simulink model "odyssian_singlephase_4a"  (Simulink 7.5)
settings: Solver=ode23t  StartTime=0.0  StopTime=6  RelTol=1e-6
undefined symbols (not defined in the file or in its folder): dfilt, DiscIntNeverNeededParam
libraries: powerlib x80, powerlib_extras x43, simulink x24, dsparch4 x4
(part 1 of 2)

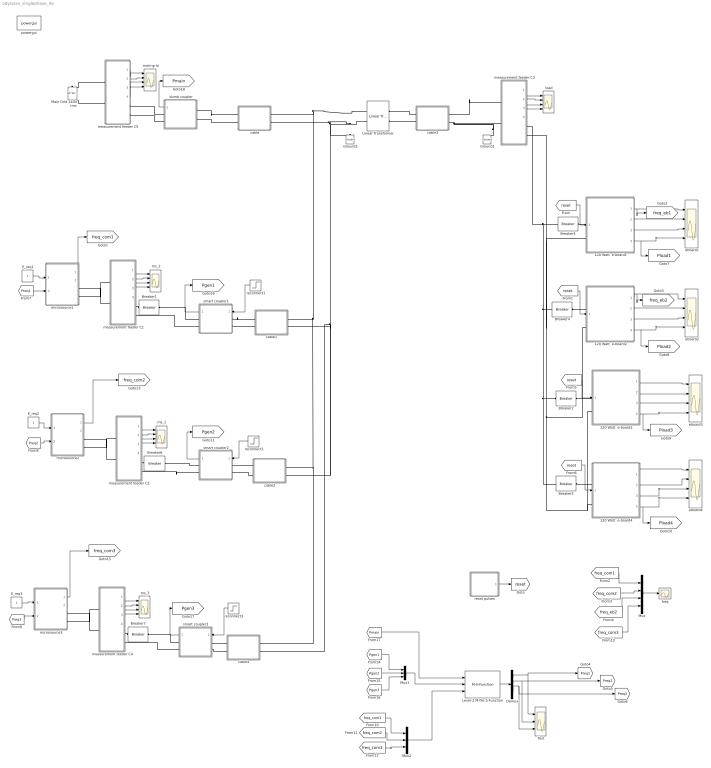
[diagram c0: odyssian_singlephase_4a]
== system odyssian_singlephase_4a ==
  " load" : Scope  NumInputPorts=4
  " main-grid" : Scope  NumInputPorts=4
  " ms_1" : Scope  NumInputPorts=4
  " ms_2" : Scope  NumInputPorts=4
  " ms_3" : Scope  NumInputPorts=4
  120 Watt  e-board1 : Subsystem  mask{tf=100, p=1}
      mask prompts: tf "fault_time"; p "load priority"
  120 Watt  e-board2 : Subsystem  mask{tf=100, p=1}
      mask prompts: tf "fault_time"; p "load priority"
  120 Watt  e-board3 : Subsystem  mask{tf=100, p=1}
      mask prompts: tf "fault_time"; p "load priority"
  120 Watt  e-board4 : Subsystem  mask{tf=100, p=2}
      mask prompts: tf "fault_time"; p "load priority"
  Breaker{1..6} (6 alike) : powerlib/Elements/Breaker  DialogController=POWERSYS.PowerSysDialog  SystemSampleTime=-1  BreakerResistance=0.01  InitialState=1  SnubberResistance=1e6  SnubberCapacitance=inf  SwitchingTimes=[100]  External=off  Measurements=None  MoreParameters=off  NoBreakLoop=off
  Breaker7 : powerlib/Elements/Breaker  DialogController=POWERSYS.PowerSysDialog  SystemSampleTime=-1  BreakerResistance=0.01  InitialState=1  SnubberResistance=1e6  SnubberCapacitance=inf  SwitchingTimes=[3 4.5]  External=off  Measurements=None  MoreParameters=off  NoBreakLoop=off
  Demux : Demux  Outputs=3
  E_req1 : Constant  OutDataType=fixdt(1, 16)  OutScaling=2^0
  E_req2 : Constant  OutDataType=fixdt(1, 16)  OutScaling=2^0
  E_req3 : Constant  OutDataType=fixdt(1, 16)  OutScaling=2^0
  Ground1 : powerlib/Elements/Ground  DialogController=POWERSYS.PowerSysDialog  PhysicalDomain=powersysdomain  SubClassName=unknown  LeftPortType=p1  RightPortType=p1  LConnTagsString=a
  Ground3 : powerlib/Elements/Ground  DialogController=POWERSYS.PowerSysDialog  PhysicalDomain=powersysdomain  SubClassName=unknown  LeftPortType=p1  RightPortType=p1  LConnTagsString=a
  Level-2 M-file S-Function : M-S-Function  FunctionName=Power_Dispatcher
  Linear Transformer : powerlib/Elements/Linear Transformer  DialogController=POWERSYS.PowerSysDialog  PhysicalDomain=powersysdomain  SubClassName=unknown  LeftPortType=p1  RightPortType=p1  LConnTagsString=a|b  RConnTagsString=A|B  UNITS=SI  NominalPower=[ 45e3 , 60 ]  winding1=[240 0.001 1.e-3]  winding2=[120 .001 1.e-3]  ThreeWindings=off  winding3=[3.15e+05 0.7938 0.084225]  RmLm=[1.0804e+06 2866]  Measurements=All voltages and currents  DataType=on
  Main Grid 240V rms : powerlib/Electrical Sources/AC Voltage Source  DialogController=POWERSYS.PowerSysDialog  SystemSampleTime=-1  Amplitude=240*sqrt(2)  Phase=0  Frequency=60  SampleTime=0  Measurements=None
  Mux : Mux
  Mux1 : Mux  Inputs=3
  Mux2 : Mux  Inputs=3
  Test : Scope  NumInputPorts=3
  cable : Subsystem
  cable1 : Subsystem
  cable2 : Subsystem
  cable3 : Subsystem
  cable4 : Subsystem
  dumb coupler : Subsystem
  eboard{1..4} (4 alike) : Scope  NumInputPorts=4
  freq : Scope
  measurement feeder C1 : Subsystem
  measurement feeder C2 : Subsystem
  measurement feeder C3 : Subsystem
  measurement feeder C4 : Subsystem
  measurement feeder C5 : Subsystem
  microsource1 : Subsystem  AncestorBlock=|
      | UWM_blocks/inverter-based
      | DG (simplified)
      | 208V - 15kVA
  microsource2 : Subsystem  AncestorBlock=|
      | UWM_blocks/inverter-based
      | DG (simplified)
      | 208V - 15kVA
  microsource3 : Subsystem  AncestorBlock=|
      | UWM_blocks/inverter-based
      | DG (simplified)
      | 208V - 15kVA
  powergui : powerlib/powergui  Priority=1  SystemSampleTime=-1  SimulationMode=Discrete  SampleTime=50e-5  frequency=60  SPID=off  DisableSnubberDevices=off  DisableRonSwitches=off  DisableVfSwitches=off  SwTol=0  Interpol=off  frequencyindice=0  echomessages=off  HookPort=off  DisplayEquations=off  FunctionMessages=off  EnableUseOfTLC=off  x0status=blocks  RestoreLinks=warning  ResistiveCurrentMeasurement=off  Frange=[0:2:500]  Ylog=off  Xlog=on  ShowGrid=off  save=off  variable=ZData  ZoomFFT=on  StartTime=0.0  cycles=1  DisplayStyle=1  fundamental=60  FreqAxis=off  MaxFrequency=1000  frequencyindicesteady=1  RmsSteady=1  display=off  Ts=0  methode=off
  reconnect1 : Step  Time=.1  SampleTime=0
  reconnect2 : Step  Time=.1  SampleTime=0
  reconnect3 : Step  Time=.1  SampleTime=0
  reset pulses : Subsystem  mask{tpulse=[50 100]}
  smart coupler1 : Subsystem
  smart coupler2 : Subsystem
  smart coupler3 : Subsystem
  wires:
  measurement feeder C3/1(Vm) -> " load"/1
  measurement feeder C3/2(Im) -> " load"/2
  measurement feeder C3/3(PQ) -> " load"/3
  measurement feeder C3/4(RMS (V-I)) -> " load"/4
  120 Watt  e-board1/1(w) -> eboard1/1, [freq_eb1]
  120 Watt  e-board1/2(Irms) -> eboard1/2
  120 Watt  e-board1/3(Vrms) -> eboard1/3
  [reset] -> 120 Watt  e-board1/1(reset)
  120 Watt  e-board2/1(w) -> eboard2/1, [freq_eb2]
  120 Watt  e-board2/2(Irms) -> eboard2/2
  120 Watt  e-board2/3(Vrms) -> eboard2/3
  [reset] -> 120 Watt  e-board2/1(reset)
  Mux/1 -> freq/1
  reset pulses/1(Out1) -> [reset]
  [freq_com1] -> Mux/1
  [freq_com2] -> Mux/2
  [freq_eb2] -> Mux/3
  measurement feeder C5/1(Vm) -> " main-grid"/1
  measurement feeder C5/2(Im) -> " main-grid"/2
  measurement feeder C5/3(PQ) -> " main-grid"/3
  measurement feeder C5/4(RMS (V-I)) -> " main-grid"/4
  measurement feeder C1/1(Vm) -> " ms_2"/1
  measurement feeder C1/2(Im) -> " ms_2"/2
  measurement feeder C1/3(PQ) -> " ms_2"/3
  measurement feeder C1/4(RMS (V-I)) -> " ms_2"/4
  E_req1/1 -> microsource1/1(E_req)
  120 Watt  e-board3/1(w) -> eboard3/1
  120 Watt  e-board3/2(Irms) -> eboard3/2
  120 Watt  e-board3/3(Vrms) -> eboard3/3
  [reset] -> 120 Watt  e-board3/1(reset)
  120 Watt  e-board4/1(w) -> eboard4/1
  120 Watt  e-board4/2(Irms) -> eboard4/2
  [reset] -> 120 Watt  e-board4/1(reset)
  measurement feeder C2/1(Vm) -> " ms_1"/1
  measurement feeder C2/2(Im) -> " ms_1"/2
  measurement feeder C2/3(PQ) -> " ms_1"/3
  measurement feeder C2/4(RMS (V-I)) -> " ms_1"/4
  E_req2/1 -> microsource2/1(E_req)
  reconnect2/1 -> smart coupler2/1(switch)
  measurement feeder C4/1(Vm) -> " ms_3"/1
  measurement feeder C4/2(Im) -> " ms_3"/2
  measurement feeder C4/3(PQ) -> " ms_3"/3
  measurement feeder C4/4(RMS (V-I)) -> " ms_3"/4
  E_req3/1 -> microsource3/1(E_req)
  [Preq2] -> microsource2/2(P_req)
  [Preq3] -> microsource3/2(P_req)
  [Preq1] -> microsource1/2(P_req)
  120 Watt  e-board1/4(Pload) -> eboard1/4, [Pload1]
  120 Watt  e-board2/4(Pload) -> eboard2/4, [Pload2]
  120 Watt  e-board3/4(Pload) -> eboard3/4, [Pload3]
  120 Watt  e-board4/3(Vrms) -> eboard4/3
  120 Watt  e-board4/4(Pload) -> eboard4/4, [Pload4]
  microsource1/1(w) -> [freq_com1]
  microsource2/1(w) -> [freq_com2]
  microsource3/1(w) -> [freq_com3]
  [Pgen2] -> Mux1/2
  smart coupler2/1(Pgen) -> [Pgen2]
  smart coupler1/1(Pgen) -> [Pgen1]
  reconnect1/1 -> smart coupler1/1(switch)
  smart coupler3/1(Pgen) -> [Pgen3]
  reconnect3/1 -> smart coupler3/1(switch)
  dumb coupler/1(Pgen) -> [Pmain]
  [Pmain] -> Level-2 M-file S-Function/1
  [Pgen1] -> Mux1/1
  [Pgen3] -> Mux1/3
  Mux1/1 -> Level-2 M-file S-Function/2
  [freq_com1] -> Mux2/1
  [freq_com2] -> Mux2/2
  [freq_com3] -> Mux2/3
  Mux2/1 -> Level-2 M-file S-Function/3
  Level-2 M-file S-Function/1 -> Demux/1
  Demux/1 -> Test/1, [Preq1]
  Demux/2 -> Test/2, [Preq2]
  Demux/3 -> Test/3, [Preq3]
  [freq_com3] -> Mux/4
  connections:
  Breaker2/RConn1 -- Breaker4/RConn1 -- measurement feeder C3/RConn1 -- Breaker3/RConn1 -- Breaker5/RConn1
  120 Watt  e-board4/LConn2 -- measurement feeder C3/RConn2 -- 120 Watt  e-board1/LConn2 -- 120 Watt  e-board2/LConn2 -- 120 Watt  e-board3/LConn2
  cable3/LConn2 -- Ground1/LConn1 -- measurement feeder C3/LConn2
  120 Watt  e-board1/LConn1 -- Breaker3/LConn1
  120 Watt  e-board2/LConn1 -- Breaker4/LConn1
  measurement feeder C5/RConn1 -- dumb coupler/RConn1
  cable4/LConn1 -- Linear Transformer/LConn1 -- cable/LConn1 -- cable1/LConn1 -- cable2/LConn1
  Linear Transformer/LConn2 -- Ground3/LConn1 -- cable2/LConn2 -- cable4/LConn2 -- cable1/LConn2 -- cable/LConn2
  cable3/LConn1 -- measurement feeder C3/LConn1
  cable3/RConn2 -- Linear Transformer/RConn2
  cable3/RConn1 -- Linear Transformer/RConn1
  measurement feeder C5/LConn1 -- Main Grid 240V rms/RConn1
  measurement feeder C5/LConn2 -- Main Grid 240V rms/LConn1
  measurement feeder C1/LConn1 -- microsource1/RConn1
  Breaker1/RConn1 -- measurement feeder C1/RConn1
  120 Watt  e-board3/LConn1 -- Breaker2/LConn1
  120 Watt  e-board4/LConn1 -- Breaker5/LConn1
  measurement feeder C2/LConn1 -- microsource2/RConn1
  measurement feeder C2/LConn2 -- microsource2/RConn2
  Breaker6/RConn1 -- measurement feeder C2/RConn1
  measurement feeder C4/LConn1 -- microsource3/RConn1
  measurement feeder C4/LConn2 -- microsource3/RConn2
  Breaker7/RConn1 -- measurement feeder C4/RConn1
  measurement feeder C1/LConn2 -- microsource1/RConn2
  cable2/RConn1 -- smart coupler2/LConn1
  cable2/RConn2 -- smart coupler2/LConn2
  smart coupler2/RConn1 -- Breaker6/LConn1
  smart coupler2/RConn2 -- measurement feeder C2/RConn2
  smart coupler1/RConn1 -- Breaker1/LConn1
  smart coupler1/LConn1 -- cable1/RConn1
  smart coupler1/LConn2 -- cable1/RConn2
  smart coupler1/RConn2 -- measurement feeder C1/RConn2
  smart coupler3/RConn1 -- Breaker7/LConn1
  smart coupler3/RConn2 -- measurement feeder C4/RConn2
  smart coupler3/LConn1 -- cable4/RConn1
  smart coupler3/LConn2 -- cable4/RConn2
  measurement feeder C5/RConn2 -- dumb coupler/RConn2
  dumb coupler/LConn1 -- cable/RConn1
  dumb coupler/LConn2 -- cable/RConn2

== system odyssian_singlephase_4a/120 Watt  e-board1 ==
  reset : Inport
  Breaker : powerlib/Elements/Breaker  DialogController=POWERSYS.PowerSysDialog  SystemSampleTime=-1  BreakerResistance=0.01  InitialState=1  SnubberResistance=1e6  SnubberCapacitance=inf  SwitchingTimes="[ 1/60  5/60 ]"  External=on  Measurements=None  MoreParameters=off  NoBreakLoop=off
  Current Measurement : powerlib/Measurements/Current Measurement  DialogController=POWERSYS.PowerSysDialog  SystemSampleTime=-1  PhasorSimulation=off  OutputType=Complex  PSBequivalent=0
  Ground : powerlib/Elements/Ground  DialogController=POWERSYS.PowerSysDialog  PhysicalDomain=powersysdomain  SubClassName=unknown  LeftPortType=p1  RightPortType=p1  LConnTagsString=a
  Product : Product  OutDataType=fixdt(1, 16)  OutScaling=2^0
  Series RLC Load : powerlib/Elements/Series RLC Load  DialogController=POWERSYS.PowerSysDialog  PhysicalDomain=powersysdomain  SubClassName=unknown  LeftPortType=p1  RightPortType=p1  LConnTagsString=a  RConnTagsString=__new0  NominalVoltage=120  NominalFrequency=60  ActivePower=120  InductivePower=0  CapacitivePower=0  Setx0=off  InitialVoltage=0  SetiL0=off  InitialCurrent=0  Measurements=None
  Voltage  Measurement : powerlib/Measurements/Voltage Measurement  DialogController=POWERSYS.PowerSysDialog  SystemSampleTime=-1  PhasorSimulation=off  OutputType=Complex  PSBequivalent=0
  trip : Subsystem  mask{p=p}
      mask prompts: p "priority level"
  A : PMIOPort  Port=1  Side=Left
  C : PMIOPort  Port=2  Side=Left
  w : Outport  OutDataType=fixdt(1, 16)  OutScaling=2^0
  Irms : Outport  Port=2  OutDataType=fixdt(1, 16)  OutScaling=2^0
  Vrms : Outport  Port=3  OutDataType=fixdt(1, 16)  OutScaling=2^0
  Pload : Outport  Port=4  OutDataType=fixdt(1, 16)  OutScaling=2^0
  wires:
  trip/1(w) -> w/1
  Current Measurement/1 -> trip/3(I)
  Voltage  Measurement/1 -> trip/2(V)
  reset/1 -> trip/1(Reset)
  trip/2(trip) -> Breaker/1
  trip/3(Irms) -> Irms/1, Product/1
  trip/4(Vrms) -> Vrms/1, Product/2
  Product/1 -> Pload/1
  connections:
  A/RConn1 -- Current Measurement/LConn1 -- Voltage  Measurement/LConn1
  Voltage  Measurement/LConn2 -- Ground/LConn1
  Current Measurement/RConn1 -- Breaker/LConn1
  Series RLC Load/LConn1 -- Breaker/RConn1
  Series RLC Load/RConn1 -- C/RConn1

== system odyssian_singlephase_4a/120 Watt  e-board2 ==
  reset : Inport
  Breaker : powerlib/Elements/Breaker  DialogController=POWERSYS.PowerSysDialog  SystemSampleTime=-1  BreakerResistance=0.01  InitialState=1  SnubberResistance=1e6  SnubberCapacitance=inf  SwitchingTimes="[ 1/60  5/60 ]"  External=on  Measurements=None  MoreParameters=off  NoBreakLoop=off
  Current Measurement : powerlib/Measurements/Current Measurement  DialogController=POWERSYS.PowerSysDialog  SystemSampleTime=-1  PhasorSimulation=off  OutputType=Complex  PSBequivalent=0
  Ground : powerlib/Elements/Ground  DialogController=POWERSYS.PowerSysDialog  PhysicalDomain=powersysdomain  SubClassName=unknown  LeftPortType=p1  RightPortType=p1  LConnTagsString=a
  Product : Product  OutDataType=fixdt(1, 16)  OutScaling=2^0
  Series RLC Load : powerlib/Elements/Series RLC Load  DialogController=POWERSYS.PowerSysDialog  PhysicalDomain=powersysdomain  SubClassName=unknown  LeftPortType=p1  RightPortType=p1  LConnTagsString=a  RConnTagsString=__new0  NominalVoltage=120  NominalFrequency=60  ActivePower=120  InductivePower=0  CapacitivePower=0  Setx0=off  InitialVoltage=0  SetiL0=off  InitialCurrent=0  Measurements=None
  Voltage  Measurement : powerlib/Measurements/Voltage Measurement  DialogController=POWERSYS.PowerSysDialog  SystemSampleTime=-1  PhasorSimulation=off  OutputType=Complex  PSBequivalent=0
  trip : Subsystem  mask{p=p}
      mask prompts: p "priority level"
  A : PMIOPort  Port=1  Side=Left
  C : PMIOPort  Port=2  Side=Left
  w : Outport  OutDataType=fixdt(1, 16)  OutScaling=2^0
  Irms : Outport  Port=2  OutDataType=fixdt(1, 16)  OutScaling=2^0
  Vrms : Outport  Port=3  OutDataType=fixdt(1, 16)  OutScaling=2^0
  Pload : Outport  Port=4  OutDataType=fixdt(1, 16)  OutScaling=2^0
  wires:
  trip/1(w) -> w/1
  Current Measurement/1 -> trip/3(I)
  Voltage  Measurement/1 -> trip/2(V)
  reset/1 -> trip/1(Reset)
  trip/2(trip) -> Breaker/1
  trip/3(Irms) -> Irms/1, Product/1
  trip/4(Vrms) -> Vrms/1, Product/2
  Product/1 -> Pload/1
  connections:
  A/RConn1 -- Current Measurement/LConn1 -- Voltage  Measurement/LConn1
  Voltage  Measurement/LConn2 -- Ground/LConn1
  Current Measurement/RConn1 -- Breaker/LConn1
  Series RLC Load/LConn1 -- Breaker/RConn1
  Series RLC Load/RConn1 -- C/RConn1

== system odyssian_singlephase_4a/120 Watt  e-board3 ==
  reset : Inport
  Breaker : powerlib/Elements/Breaker  DialogController=POWERSYS.PowerSysDialog  SystemSampleTime=-1  BreakerResistance=0.01  InitialState=1  SnubberResistance=1e6  SnubberCapacitance=inf  SwitchingTimes="[ 1/60  5/60 ]"  External=on  Measurements=None  MoreParameters=off  NoBreakLoop=off
  Current Measurement : powerlib/Measurements/Current Measurement  DialogController=POWERSYS.PowerSysDialog  SystemSampleTime=-1  PhasorSimulation=off  OutputType=Complex  PSBequivalent=0
  Ground : powerlib/Elements/Ground  DialogController=POWERSYS.PowerSysDialog  PhysicalDomain=powersysdomain  SubClassName=unknown  LeftPortType=p1  RightPortType=p1  LConnTagsString=a
  Product : Product  OutDataType=fixdt(1, 16)  OutScaling=2^0
  Series RLC Load : powerlib/Elements/Series RLC Load  DialogController=POWERSYS.PowerSysDialog  PhysicalDomain=powersysdomain  SubClassName=unknown  LeftPortType=p1  RightPortType=p1  LConnTagsString=a  RConnTagsString=__new0  NominalVoltage=120  NominalFrequency=60  ActivePower=120  InductivePower=0  CapacitivePower=0  Setx0=off  InitialVoltage=0  SetiL0=off  InitialCurrent=0  Measurements=None
  Voltage  Measurement : powerlib/Measurements/Voltage Measurement  DialogController=POWERSYS.PowerSysDialog  SystemSampleTime=-1  PhasorSimulation=off  OutputType=Complex  PSBequivalent=0
  trip : Subsystem  mask{p=p}
      mask prompts: p "priority level"
  A : PMIOPort  Port=1  Side=Left
  C : PMIOPort  Port=2  Side=Left
  w : Outport  OutDataType=fixdt(1, 16)  OutScaling=2^0
  Irms : Outport  Port=2  OutDataType=fixdt(1, 16)  OutScaling=2^0
  Vrms : Outport  Port=3  OutDataType=fixdt(1, 16)  OutScaling=2^0
  Pload : Outport  Port=4  OutDataType=fixdt(1, 16)  OutScaling=2^0
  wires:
  trip/1(w) -> w/1
  Current Measurement/1 -> trip/3(I)
  Voltage  Measurement/1 -> trip/2(V)
  reset/1 -> trip/1(Reset)
  trip/2(trip) -> Breaker/1
  trip/3(Irms) -> Irms/1, Product/1
  trip/4(Vrms) -> Vrms/1, Product/2
  Product/1 -> Pload/1
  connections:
  A/RConn1 -- Current Measurement/LConn1 -- Voltage  Measurement/LConn1
  Voltage  Measurement/LConn2 -- Ground/LConn1
  Current Measurement/RConn1 -- Breaker/LConn1
  Series RLC Load/LConn1 -- Breaker/RConn1
  Series RLC Load/RConn1 -- C/RConn1

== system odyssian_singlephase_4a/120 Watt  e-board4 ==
  reset : Inport
  Breaker : powerlib/Elements/Breaker  DialogController=POWERSYS.PowerSysDialog  SystemSampleTime=-1  BreakerResistance=0.01  InitialState=1  SnubberResistance=1e6  SnubberCapacitance=inf  SwitchingTimes="[ 1/60  5/60 ]"  External=on  Measurements=None  MoreParameters=off  NoBreakLoop=off
  Current Measurement : powerlib/Measurements/Current Measurement  DialogController=POWERSYS.PowerSysDialog  SystemSampleTime=-1  PhasorSimulation=off  OutputType=Complex  PSBequivalent=0
  Ground : powerlib/Elements/Ground  DialogController=POWERSYS.PowerSysDialog  PhysicalDomain=powersysdomain  SubClassName=unknown  LeftPortType=p1  RightPortType=p1  LConnTagsString=a
  Product : Product  OutDataType=fixdt(1, 16)  OutScaling=2^0
  Series RLC Load : powerlib/Elements/Series RLC Load  DialogController=POWERSYS.PowerSysDialog  PhysicalDomain=powersysdomain  SubClassName=unknown  LeftPortType=p1  RightPortType=p1  LConnTagsString=a  RConnTagsString=__new0  NominalVoltage=120  NominalFrequency=60  ActivePower=120  InductivePower=0  CapacitivePower=0  Setx0=off  InitialVoltage=0  SetiL0=off  InitialCurrent=0  Measurements=None
  Voltage  Measurement : powerlib/Measurements/Voltage Measurement  DialogController=POWERSYS.PowerSysDialog  SystemSampleTime=-1  PhasorSimulation=off  OutputType=Complex  PSBequivalent=0
  trip : Subsystem  mask{p=p}
      mask prompts: p "priority level"
  A : PMIOPort  Port=1  Side=Left
  C : PMIOPort  Port=2  Side=Left
  w : Outport  OutDataType=fixdt(1, 16)  OutScaling=2^0
  Irms : Outport  Port=2  OutDataType=fixdt(1, 16)  OutScaling=2^0
  Vrms : Outport  Port=3  OutDataType=fixdt(1, 16)  OutScaling=2^0
  Pload : Outport  Port=4  OutDataType=fixdt(1, 16)  OutScaling=2^0
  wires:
  trip/1(w) -> w/1
  Current Measurement/1 -> trip/3(I)
  Voltage  Measurement/1 -> trip/2(V)
  reset/1 -> trip/1(Reset)
  trip/2(trip) -> Breaker/1
  trip/3(Irms) -> Irms/1, Product/1
  trip/4(Vrms) -> Vrms/1, Product/2
  Product/1 -> Pload/1
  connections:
  A/RConn1 -- Current Measurement/LConn1 -- Voltage  Measurement/LConn1
  Voltage  Measurement/LConn2 -- Ground/LConn1
  Current Measurement/RConn1 -- Breaker/LConn1
  Series RLC Load/LConn1 -- Breaker/RConn1
  Series RLC Load/RConn1 -- C/RConn1

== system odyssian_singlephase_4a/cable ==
  Series RLC Branch : powerlib/Elements/Series RLC Branch  DialogController=POWERSYS.PowerSysDialog  PhysicalDomain=powersysdomain  SubClassName=unknown  LeftPortType=p1  RightPortType=p1  LConnTagsString=__new0  RConnTagsString=__new0  BranchType=RL  Resistance=.001  Inductance=1.e-5  SetiL0=off  InitialCurrent=0  Capacitance=1e-6  Setx0=off  InitialVoltage=0  Measurements=None
  A : PMIOPort  Tag=PMCPort  Port=1  Side=Left
  A' : PMIOPort  Tag=PMCPort  Port=2  Side=Right
  B' : PMIOPort  Tag=PMCPort  Port=3  Side=Right
  B : PMIOPort  Tag=PMCPort  Port=4  Side=Left
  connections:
  A/RConn1 -- Series RLC Branch/LConn1
  A'/RConn1 -- Series RLC Branch/RConn1
  B/RConn1 -- B'/RConn1

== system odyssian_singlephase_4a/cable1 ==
  Series RLC Branch : powerlib/Elements/Series RLC Branch  DialogController=POWERSYS.PowerSysDialog  PhysicalDomain=powersysdomain  SubClassName=unknown  LeftPortType=p1  RightPortType=p1  LConnTagsString=__new0  RConnTagsString=__new0  BranchType=RL  Resistance=.001  Inductance=1.e-6  SetiL0=off  InitialCurrent=0  Capacitance=1e-6  Setx0=off  InitialVoltage=0  Measurements=None
  A : PMIOPort  Tag=PMCPort  Port=1  Side=Left
  A' : PMIOPort  Tag=PMCPort  Port=2  Side=Right
  B' : PMIOPort  Tag=PMCPort  Port=3  Side=Right
  B : PMIOPort  Tag=PMCPort  Port=4  Side=Left
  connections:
  A/RConn1 -- Series RLC Branch/LConn1
  Series RLC Branch/RConn1 -- A'/RConn1
  B/RConn1 -- B'/RConn1

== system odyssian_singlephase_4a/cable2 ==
  Series RLC Branch : powerlib/Elements/Series RLC Branch  DialogController=POWERSYS.PowerSysDialog  PhysicalDomain=powersysdomain  SubClassName=unknown  LeftPortType=p1  RightPortType=p1  LConnTagsString=__new0  RConnTagsString=__new0  BranchType=RL  Resistance=.001  Inductance=1.e-6  SetiL0=off  InitialCurrent=0  Capacitance=1e-6  Setx0=off  InitialVoltage=0  Measurements=None
  A : PMIOPort  Tag=PMCPort  Port=1  Side=Left
  A' : PMIOPort  Tag=PMCPort  Port=2  Side=Right
  B' : PMIOPort  Tag=PMCPort  Port=3  Side=Right
  B : PMIOPort  Tag=PMCPort  Port=4  Side=Left
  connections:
  A/RConn1 -- Series RLC Branch/LConn1
  Series RLC Branch/RConn1 -- A'/RConn1
  B/RConn1 -- B'/RConn1

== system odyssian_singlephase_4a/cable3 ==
  Series RLC Branch : powerlib/Elements/Series RLC Branch  DialogController=POWERSYS.PowerSysDialog  PhysicalDomain=powersysdomain  SubClassName=unknown  LeftPortType=p1  RightPortType=p1  LConnTagsString=__new0  RConnTagsString=__new0  BranchType=RL  Resistance=.001  Inductance=1.e-6  SetiL0=off  InitialCurrent=0  Capacitance=1e-6  Setx0=off  InitialVoltage=0  Measurements=None
  A : PMIOPort  Tag=PMCPort  Port=1  Side=Left
  A' : PMIOPort  Tag=PMCPort  Port=2  Side=Right
  B' : PMIOPort  Tag=PMCPort  Port=3  Side=Right
  B : PMIOPort  Tag=PMCPort  Port=4  Side=Left
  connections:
  A/RConn1 -- Series RLC Branch/LConn1
  Series RLC Branch/RConn1 -- A'/RConn1
  B/RConn1 -- B'/RConn1

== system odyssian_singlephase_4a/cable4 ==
  Series RLC Branch : powerlib/Elements/Series RLC Branch  DialogController=POWERSYS.PowerSysDialog  PhysicalDomain=powersysdomain  SubClassName=unknown  LeftPortType=p1  RightPortType=p1  LConnTagsString=__new0  RConnTagsString=__new0  BranchType=RL  Resistance=.001  Inductance=1.e-6  SetiL0=off  InitialCurrent=0  Capacitance=1e-6  Setx0=off  InitialVoltage=0  Measurements=None
  A : PMIOPort  Tag=PMCPort  Port=1  Side=Left
  A' : PMIOPort  Tag=PMCPort  Port=2  Side=Right
  B' : PMIOPort  Tag=PMCPort  Port=3  Side=Right
  B : PMIOPort  Tag=PMCPort  Port=4  Side=Left
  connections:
  A/RConn1 -- Series RLC Branch/LConn1
  Series RLC Branch/RConn1 -- A'/RConn1
  B/RConn1 -- B'/RConn1

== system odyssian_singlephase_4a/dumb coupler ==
  Breaker : powerlib/Elements/Breaker  DialogController=POWERSYS.PowerSysDialog  SystemSampleTime=-1  BreakerResistance=0.01  InitialState=1  SnubberResistance=1e6  SnubberCapacitance=inf  SwitchingTimes=[ 2 ]  External=off  Measurements=None  MoreParameters=off  NoBreakLoop=off
  Current Measurement : powerlib/Measurements/Current Measurement  DialogController=POWERSYS.PowerSysDialog  SystemSampleTime=-1  PhasorSimulation=off  OutputType=Complex  PSBequivalent=0
  Product : Product  OutDataType=fixdt(1, 16)  OutScaling=2^0
  "RMS " : powerlib_extras/Measurements/RMS  DialogController=POWERSYS.PowerSysDialog  SystemSampleTime=-1  f1=60
  RMS 1 : powerlib_extras/Measurements/RMS  DialogController=POWERSYS.PowerSysDialog  SystemSampleTime=-1  f1=60
  Voltage Measurement1 : powerlib/Measurements/Voltage Measurement  DialogController=POWERSYS.PowerSysDialog  SystemSampleTime=-1  PhasorSimulation=off  OutputType=Complex  PSBequivalent=0
  A : PMIOPort  Port=1  Side=Left
  C : PMIOPort  Port=2  Side=Left
  a : PMIOPort  Port=3  Side=Right
  c : PMIOPort  Port=4  Side=Right
  Pgen : Outport  OutDataType=fixdt(1, 16)  OutScaling=2^0
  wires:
  "RMS "/1 -> Product/1
  RMS 1/1 -> Product/2
  Product/1 -> Pgen/1
  Current Measurement/1 -> "RMS "/1
  Voltage Measurement1/1 -> RMS 1/1
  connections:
  Breaker/LConn1 -- Current Measurement/LConn1 -- Voltage Measurement1/LConn1
  a/RConn1 -- Breaker/RConn1
  c/RConn1 -- C/RConn1 -- Voltage Measurement1/LConn2
  Current Measurement/RConn1 -- A/RConn1

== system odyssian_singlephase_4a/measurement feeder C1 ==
  Active & Reactive Power : powerlib_extras/Measurements/Active & Reactive Power  DialogController=POWERSYS.PowerSysDialog  SystemSampleTime=-1  f1=60
  Current Measurement : powerlib/Measurements/Current Measurement  DialogController=POWERSYS.PowerSysDialog  SystemSampleTime=-1  PhasorSimulation=off  OutputType=Complex  PSBequivalent=0
  Mux : Mux  Inputs=2
  RMS : powerlib_extras/Measurements/RMS  DialogController=POWERSYS.PowerSysDialog  SystemSampleTime=-1  f1=60
  RMS1 : powerlib_extras/Measurements/RMS  DialogController=POWERSYS.PowerSysDialog  SystemSampleTime=-1  f1=60
  Voltage Measurement : powerlib/Measurements/Voltage Measurement  DialogController=POWERSYS.PowerSysDialog  SystemSampleTime=-1  PhasorSimulation=off  OutputType=Complex  PSBequivalent=0
  A : PMIOPort  Port=1  Side=Left
  a : PMIOPort  Port=2  Side=Right
  GND : PMIOPort  Port=3  Side=Left
  c : PMIOPort  Port=4  Side=Right
  Vm : Outport  OutDataType=fixdt(1, 16)  OutScaling=2^0
  Im : Outport  Port=2  OutDataType=fixdt(1, 16)  OutScaling=2^0
  PQ : Outport  Port=3  OutDataType=fixdt(1, 16)  OutScaling=2^0
  RMS (V-I) : Outport  Port=4  OutDataType=fixdt(1, 16)  OutScaling=2^0
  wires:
  Mux/1 -> RMS (V-I)/1
  Current Measurement/1 -> Im/1, RMS1/1, Active & Reactive Power/2
  Voltage Measurement/1 -> Vm/1, RMS/1, Active & Reactive Power/1
  Active & Reactive Power/1 -> PQ/1
  RMS/1 -> Mux/1
  RMS1/1 -> Mux/2
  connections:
  a/RConn1 -- Current Measurement/RConn1
  Voltage Measurement/LConn1 -- A/RConn1 -- Current Measurement/LConn1
  Voltage Measurement/LConn2 -- GND/RConn1 -- c/RConn1

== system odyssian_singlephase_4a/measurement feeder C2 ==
  Active & Reactive Power : powerlib_extras/Measurements/Active & Reactive Power  DialogController=POWERSYS.PowerSysDialog  SystemSampleTime=-1  f1=60
  Current Measurement : powerlib/Measurements/Current Measurement  DialogController=POWERSYS.PowerSysDialog  SystemSampleTime=-1  PhasorSimulation=off  OutputType=Complex  PSBequivalent=0
  Mux : Mux  Inputs=2
  RMS : powerlib_extras/Measurements/RMS  DialogController=POWERSYS.PowerSysDialog  SystemSampleTime=-1  f1=60
  RMS1 : powerlib_extras/Measurements/RMS  DialogController=POWERSYS.PowerSysDialog  SystemSampleTime=-1  f1=60
  Voltage Measurement : powerlib/Measurements/Voltage Measurement  DialogController=POWERSYS.PowerSysDialog  SystemSampleTime=-1  PhasorSimulation=off  OutputType=Complex  PSBequivalent=0
  A : PMIOPort  Port=1  Side=Left
  a : PMIOPort  Port=2  Side=Right
  GND : PMIOPort  Port=3  Side=Left
  c : PMIOPort  Port=4  Side=Right
  Vm : Outport  OutDataType=fixdt(1, 16)  OutScaling=2^0
  Im : Outport  Port=2  OutDataType=fixdt(1, 16)  OutScaling=2^0
  PQ : Outport  Port=3  OutDataType=fixdt(1, 16)  OutScaling=2^0
  RMS (V-I) : Outport  Port=4  OutDataType=fixdt(1, 16)  OutScaling=2^0
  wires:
  Mux/1 -> RMS (V-I)/1
  Current Measurement/1 -> Im/1, RMS1/1, Active & Reactive Power/2
  Voltage Measurement/1 -> Vm/1, RMS/1, Active & Reactive Power/1
  Active & Reactive Power/1 -> PQ/1
  RMS/1 -> Mux/1
  RMS1/1 -> Mux/2
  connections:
  a/RConn1 -- Current Measurement/RConn1
  Voltage Measurement/LConn1 -- A/RConn1 -- Current Measurement/LConn1
  Voltage Measurement/LConn2 -- GND/RConn1 -- c/RConn1

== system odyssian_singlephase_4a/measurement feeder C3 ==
  Active & Reactive Power : powerlib_extras/Measurements/Active & Reactive Power  DialogController=POWERSYS.PowerSysDialog  SystemSampleTime=-1  f1=60
  Current Measurement : powerlib/Measurements/Current Measurement  DialogController=POWERSYS.PowerSysDialog  SystemSampleTime=-1  PhasorSimulation=off  OutputType=Complex  PSBequivalent=0
  Mux : Mux  Inputs=2
  RMS : powerlib_extras/Measurements/RMS  DialogController=POWERSYS.PowerSysDialog  SystemSampleTime=-1  f1=60
  RMS1 : powerlib_extras/Measurements/RMS  DialogController=POWERSYS.PowerSysDialog  SystemSampleTime=-1  f1=60
  Voltage Measurement : powerlib/Measurements/Voltage Measurement  DialogController=POWERSYS.PowerSysDialog  SystemSampleTime=-1  PhasorSimulation=off  OutputType=Complex  PSBequivalent=0
  A : PMIOPort  Port=1  Side=Left
  a : PMIOPort  Port=2  Side=Right
  GND : PMIOPort  Port=3  Side=Left
  c : PMIOPort  Port=4  Side=Right
  Vm : Outport  OutDataType=fixdt(1, 16)  OutScaling=2^0
  Im : Outport  Port=2  OutDataType=fixdt(1, 16)  OutScaling=2^0
  PQ : Outport  Port=3  OutDataType=fixdt(1, 16)  OutScaling=2^0
  RMS (V-I) : Outport  Port=4  OutDataType=fixdt(1, 16)  OutScaling=2^0
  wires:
  Mux/1 -> RMS (V-I)/1
  Current Measurement/1 -> Im/1, RMS1/1, Active & Reactive Power/2
  Voltage Measurement/1 -> Vm/1, RMS/1, Active & Reactive Power/1
  Active & Reactive Power/1 -> PQ/1
  RMS/1 -> Mux/1
  RMS1/1 -> Mux/2
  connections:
  a/RConn1 -- Current Measurement/RConn1
  Voltage Measurement/LConn1 -- A/RConn1 -- Current Measurement/LConn1
  Voltage Measurement/LConn2 -- GND/RConn1 -- c/RConn1

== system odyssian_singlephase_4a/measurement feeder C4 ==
  Active & Reactive Power : powerlib_extras/Measurements/Active & Reactive Power  DialogController=POWERSYS.PowerSysDialog  SystemSampleTime=-1  f1=60
  Current Measurement : powerlib/Measurements/Current Measurement  DialogController=POWERSYS.PowerSysDialog  SystemSampleTime=-1  PhasorSimulation=off  OutputType=Complex  PSBequivalent=0
  Mux : Mux  Inputs=2
  RMS : powerlib_extras/Measurements/RMS  DialogController=POWERSYS.PowerSysDialog  SystemSampleTime=-1  f1=60
  RMS1 : powerlib_extras/Measurements/RMS  DialogController=POWERSYS.PowerSysDialog  SystemSampleTime=-1  f1=60
  Voltage Measurement : powerlib/Measurements/Voltage Measurement  DialogController=POWERSYS.PowerSysDialog  SystemSampleTime=-1  PhasorSimulation=off  OutputType=Complex  PSBequivalent=0
  A : PMIOPort  Port=1  Side=Left
  a : PMIOPort  Port=2  Side=Right
  GND : PMIOPort  Port=3  Side=Left
  c : PMIOPort  Port=4  Side=Right
  Vm : Outport  OutDataType=fixdt(1, 16)  OutScaling=2^0
  Im : Outport  Port=2  OutDataType=fixdt(1, 16)  OutScaling=2^0
  PQ : Outport  Port=3  OutDataType=fixdt(1, 16)  OutScaling=2^0
  RMS (V-I) : Outport  Port=4  OutDataType=fixdt(1, 16)  OutScaling=2^0
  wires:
  Mux/1 -> RMS (V-I)/1
  Current Measurement/1 -> Im/1, RMS1/1, Active & Reactive Power/2
  Voltage Measurement/1 -> Vm/1, RMS/1, Active & Reactive Power/1
  Active & Reactive Power/1 -> PQ/1
  RMS/1 -> Mux/1
  RMS1/1 -> Mux/2
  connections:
  a/RConn1 -- Current Measurement/RConn1
  Voltage Measurement/LConn1 -- A/RConn1 -- Current Measurement/LConn1
  Voltage Measurement/LConn2 -- GND/RConn1 -- c/RConn1

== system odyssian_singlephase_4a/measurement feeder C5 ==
  Active & Reactive Power : powerlib_extras/Measurements/Active & Reactive Power  DialogController=POWERSYS.PowerSysDialog  SystemSampleTime=-1  f1=60
  Current Measurement : powerlib/Measurements/Current Measurement  DialogController=POWERSYS.PowerSysDialog  SystemSampleTime=-1  PhasorSimulation=off  OutputType=Complex  PSBequivalent=0
  Mux : Mux  Inputs=2
  RMS : powerlib_extras/Measurements/RMS  DialogController=POWERSYS.PowerSysDialog  SystemSampleTime=-1  f1=60
  RMS1 : powerlib_extras/Measurements/RMS  DialogController=POWERSYS.PowerSysDialog  SystemSampleTime=-1  f1=60
  Voltage Measurement : powerlib/Measurements/Voltage Measurement  DialogController=POWERSYS.PowerSysDialog  SystemSampleTime=-1  PhasorSimulation=off  OutputType=Complex  PSBequivalent=0
  A : PMIOPort  Port=1  Side=Left
  a : PMIOPort  Port=2  Side=Right
  GND : PMIOPort  Port=3  Side=Left
  c : PMIOPort  Port=4  Side=Right
  Vm : Outport  OutDataType=fixdt(1, 16)  OutScaling=2^0
  Im : Outport  Port=2  OutDataType=fixdt(1, 16)  OutScaling=2^0
  PQ : Outport  Port=3  OutDataType=fixdt(1, 16)  OutScaling=2^0
  RMS (V-I) : Outport  Port=4  OutDataType=fixdt(1, 16)  OutScaling=2^0
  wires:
  Mux/1 -> RMS (V-I)/1
  Current Measurement/1 -> Im/1, RMS1/1, Active & Reactive Power/2
  Voltage Measurement/1 -> Vm/1, RMS/1, Active & Reactive Power/1
  Active & Reactive Power/1 -> PQ/1
  RMS/1 -> Mux/1
  RMS1/1 -> Mux/2
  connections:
  a/RConn1 -- Current Measurement/RConn1
  Voltage Measurement/LConn1 -- A/RConn1 -- Current Measurement/LConn1
  Voltage Measurement/LConn2 -- GND/RConn1 -- c/RConn1

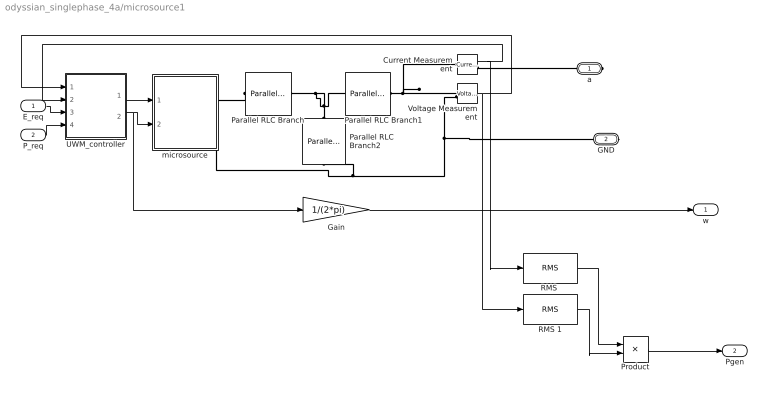
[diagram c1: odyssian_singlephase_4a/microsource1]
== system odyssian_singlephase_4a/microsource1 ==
  E_req : Inport
  P_req : Inport  Port=2
  Current Measurement : powerlib/Measurements/Current Measurement  DialogController=POWERSYS.PowerSysDialog  SystemSampleTime=-1  PhasorSimulation=off  OutputType=Complex  PSBequivalent=0
  Gain : Gain  Gain=1/(2*pi)  ParameterDataType=fixdt(1, 16)  ParameterScaling=2^0  OutDataType=fixdt(1, 16)  OutScaling=2^0
  Parallel RLC Branch : powerlib/Elements/Parallel RLC Branch  DialogController=POWERSYS.PowerSysDialog  PhysicalDomain=powersysdomain  SubClassName=unknown  LeftPortType=p1  RightPortType=p1  LConnTagsString=a  RConnTagsString=__new0  BranchType=L  Resistance=1  Inductance=1.e-1  SetiL0=off  InitialCurrent=0  Capacitance=1e-6  Setx0=off  InitialVoltage=0  Measurements=None
  Parallel RLC Branch1 : powerlib/Elements/Parallel RLC Branch  DialogController=POWERSYS.PowerSysDialog  PhysicalDomain=powersysdomain  SubClassName=unknown  LeftPortType=p1  RightPortType=p1  LConnTagsString=a  RConnTagsString=__new0  BranchType=L  Resistance=1  Inductance=1.e-1  SetiL0=off  InitialCurrent=0  Capacitance=1e-6  Setx0=off  InitialVoltage=0  Measurements=None
  Parallel RLC Branch2 : powerlib/Elements/Parallel RLC Branch  DialogController=POWERSYS.PowerSysDialog  PhysicalDomain=powersysdomain  SubClassName=unknown  LeftPortType=p1  RightPortType=p1  LConnTagsString=a  RConnTagsString=__new0  BranchType=C  Resistance=1  Inductance=1.e-1  SetiL0=off  InitialCurrent=0  Capacitance=1.e-5  Setx0=off  InitialVoltage=0  Measurements=None
  Product : Product  OutDataType=fixdt(1, 16)  OutScaling=2^0
  "RMS " : powerlib_extras/Measurements/RMS  DialogController=POWERSYS.PowerSysDialog  SystemSampleTime=-1  f1=60
  RMS 1 : powerlib_extras/Measurements/RMS  DialogController=POWERSYS.PowerSysDialog  SystemSampleTime=-1  f1=60
  UWM_controller : Subsystem  mask{Vbase=240*sqrt(2), Sbase=200}
  Voltage Measurement : powerlib/Measurements/Voltage Measurement  DialogController=POWERSYS.PowerSysDialog  SystemSampleTime=-1  PhasorSimulation=off  OutputType=Complex  PSBequivalent=0
  microsource : Subsystem
  a : PMIOPort  Port=1  Side=Right
  GND : PMIOPort  Port=2  Side=Right
  w : Outport  OutDataType=fixdt(1, 16)  OutScaling=2^0
  Pgen : Outport  Port=2  OutDataType=fixdt(1, 16)  OutScaling=2^0
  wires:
  E_req/1 -> UWM_controller/3(E_req)
  P_req/1 -> UWM_controller/4(P_req)
  UWM_controller/1(Vpk) -> microsource/1(Vpk)
  UWM_controller/2(w) -> microsource/2(w), Gain/1
  Current Measurement/1 -> UWM_controller/2(i_meas), "RMS "/1
  Voltage Measurement/1 -> UWM_controller/1(v_meas), RMS 1/1
  "RMS "/1 -> Product/1
  RMS 1/1 -> Product/2
  Gain/1 -> w/1
  Product/1 -> Pgen/1
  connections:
  Voltage Measurement/LConn2 -- GND/RConn1 -- Parallel RLC Branch2/RConn1 -- microsource/RConn2
  Parallel RLC Branch1/RConn1 -- Voltage Measurement/LConn1 -- Current Measurement/LConn1
  a/RConn1 -- Current Measurement/RConn1
  Parallel RLC Branch/LConn1 -- microsource/RConn1
  Parallel RLC Branch2/LConn1 -- Parallel RLC Branch1/LConn1 -- Parallel RLC Branch/RConn1

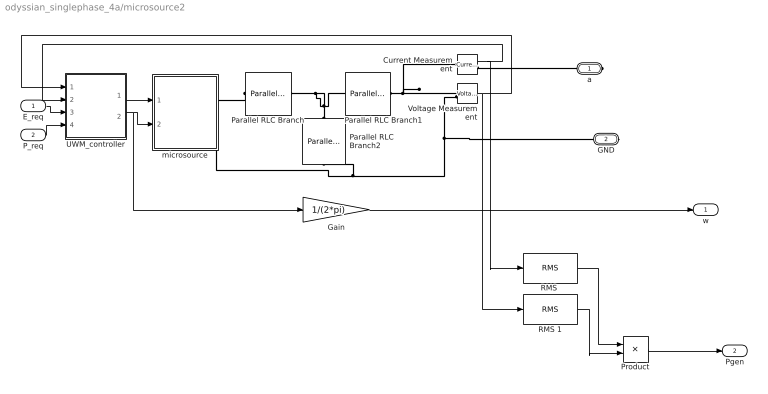
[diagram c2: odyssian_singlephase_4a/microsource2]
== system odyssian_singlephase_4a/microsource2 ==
  E_req : Inport
  P_req : Inport  Port=2
  Current Measurement : powerlib/Measurements/Current Measurement  DialogController=POWERSYS.PowerSysDialog  SystemSampleTime=-1  PhasorSimulation=off  OutputType=Complex  PSBequivalent=0
  Gain : Gain  Gain=1/(2*pi)  ParameterDataType=fixdt(1, 16)  ParameterScaling=2^0  OutDataType=fixdt(1, 16)  OutScaling=2^0
  Parallel RLC Branch : powerlib/Elements/Parallel RLC Branch  DialogController=POWERSYS.PowerSysDialog  PhysicalDomain=powersysdomain  SubClassName=unknown  LeftPortType=p1  RightPortType=p1  LConnTagsString=a  RConnTagsString=__new0  BranchType=L  Resistance=1  Inductance=1.e-1  SetiL0=off  InitialCurrent=0  Capacitance=1e-6  Setx0=off  InitialVoltage=0  Measurements=None
  Parallel RLC Branch1 : powerlib/Elements/Parallel RLC Branch  DialogController=POWERSYS.PowerSysDialog  PhysicalDomain=powersysdomain  SubClassName=unknown  LeftPortType=p1  RightPortType=p1  LConnTagsString=a  RConnTagsString=__new0  BranchType=L  Resistance=1  Inductance=1.e-1  SetiL0=off  InitialCurrent=0  Capacitance=1e-6  Setx0=off  InitialVoltage=0  Measurements=None
  Parallel RLC Branch2 : powerlib/Elements/Parallel RLC Branch  DialogController=POWERSYS.PowerSysDialog  PhysicalDomain=powersysdomain  SubClassName=unknown  LeftPortType=p1  RightPortType=p1  LConnTagsString=a  RConnTagsString=__new0  BranchType=C  Resistance=1  Inductance=1.e-1  SetiL0=off  InitialCurrent=0  Capacitance=1.e-5  Setx0=off  InitialVoltage=0  Measurements=None
  Product : Product  OutDataType=fixdt(1, 16)  OutScaling=2^0
  "RMS " : powerlib_extras/Measurements/RMS  DialogController=POWERSYS.PowerSysDialog  SystemSampleTime=-1  f1=60
  RMS 1 : powerlib_extras/Measurements/RMS  DialogController=POWERSYS.PowerSysDialog  SystemSampleTime=-1  f1=60
  UWM_controller : Subsystem  mask{Vbase=240*sqrt(2), Sbase=200}
  Voltage Measurement : powerlib/Measurements/Voltage Measurement  DialogController=POWERSYS.PowerSysDialog  SystemSampleTime=-1  PhasorSimulation=off  OutputType=Complex  PSBequivalent=0
  microsource : Subsystem
  a : PMIOPort  Port=1  Side=Right
  GND : PMIOPort  Port=2  Side=Right
  w : Outport  OutDataType=fixdt(1, 16)  OutScaling=2^0
  Pgen : Outport  Port=2  OutDataType=fixdt(1, 16)  OutScaling=2^0
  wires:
  E_req/1 -> UWM_controller/3(E_req)
  P_req/1 -> UWM_controller/4(P_req)
  UWM_controller/1(Vpk) -> microsource/1(Vpk)
  UWM_controller/2(w) -> microsource/2(w), Gain/1
  Current Measurement/1 -> UWM_controller/2(i_meas), "RMS "/1
  Voltage Measurement/1 -> UWM_controller/1(v_meas), RMS 1/1
  "RMS "/1 -> Product/1
  RMS 1/1 -> Product/2
  Gain/1 -> w/1
  Product/1 -> Pgen/1
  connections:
  Voltage Measurement/LConn2 -- GND/RConn1 -- Parallel RLC Branch2/RConn1 -- microsource/RConn2
  Parallel RLC Branch1/RConn1 -- Voltage Measurement/LConn1 -- Current Measurement/LConn1
  a/RConn1 -- Current Measurement/RConn1
  Parallel RLC Branch/LConn1 -- microsource/RConn1
  Parallel RLC Branch2/LConn1 -- Parallel RLC Branch1/LConn1 -- Parallel RLC Branch/RConn1

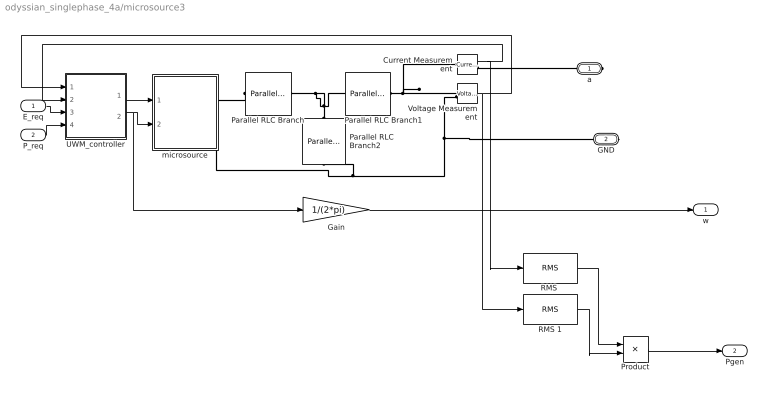
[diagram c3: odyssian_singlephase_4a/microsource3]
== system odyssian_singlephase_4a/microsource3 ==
  E_req : Inport
  P_req : Inport  Port=2
  Current Measurement : powerlib/Measurements/Current Measurement  DialogController=POWERSYS.PowerSysDialog  SystemSampleTime=-1  PhasorSimulation=off  OutputType=Complex  PSBequivalent=0
  Gain : Gain  Gain=1/(2*pi)  ParameterDataType=fixdt(1, 16)  ParameterScaling=2^0  OutDataType=fixdt(1, 16)  OutScaling=2^0
  Parallel RLC Branch : powerlib/Elements/Parallel RLC Branch  DialogController=POWERSYS.PowerSysDialog  PhysicalDomain=powersysdomain  SubClassName=unknown  LeftPortType=p1  RightPortType=p1  LConnTagsString=a  RConnTagsString=__new0  BranchType=L  Resistance=1  Inductance=1.e-1  SetiL0=off  InitialCurrent=0  Capacitance=1e-6  Setx0=off  InitialVoltage=0  Measurements=None
  Parallel RLC Branch1 : powerlib/Elements/Parallel RLC Branch  DialogController=POWERSYS.PowerSysDialog  PhysicalDomain=powersysdomain  SubClassName=unknown  LeftPortType=p1  RightPortType=p1  LConnTagsString=a  RConnTagsString=__new0  BranchType=L  Resistance=1  Inductance=1.e-1  SetiL0=off  InitialCurrent=0  Capacitance=1e-6  Setx0=off  InitialVoltage=0  Measurements=None
  Parallel RLC Branch2 : powerlib/Elements/Parallel RLC Branch  DialogController=POWERSYS.PowerSysDialog  PhysicalDomain=powersysdomain  SubClassName=unknown  LeftPortType=p1  RightPortType=p1  LConnTagsString=a  RConnTagsString=__new0  BranchType=C  Resistance=1  Inductance=1.e-1  SetiL0=off  InitialCurrent=0  Capacitance=1.e-5  Setx0=off  InitialVoltage=0  Measurements=None
  Product : Product  OutDataType=fixdt(1, 16)  OutScaling=2^0
  "RMS " : powerlib_extras/Measurements/RMS  DialogController=POWERSYS.PowerSysDialog  SystemSampleTime=-1  f1=60
  RMS 1 : powerlib_extras/Measurements/RMS  DialogController=POWERSYS.PowerSysDialog  SystemSampleTime=-1  f1=60
  UWM_controller : Subsystem  mask{Vbase=240*sqrt(2), Sbase=200}
  Voltage Measurement : powerlib/Measurements/Voltage Measurement  DialogController=POWERSYS.PowerSysDialog  SystemSampleTime=-1  PhasorSimulation=off  OutputType=Complex  PSBequivalent=0
  microsource : Subsystem
  a : PMIOPort  Port=1  Side=Right
  GND : PMIOPort  Port=2  Side=Right
  w : Outport  OutDataType=fixdt(1, 16)  OutScaling=2^0
  Pgen : Outport  Port=2  OutDataType=fixdt(1, 16)  OutScaling=2^0
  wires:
  E_req/1 -> UWM_controller/3(E_req)
  P_req/1 -> UWM_controller/4(P_req)
  UWM_controller/1(Vpk) -> microsource/1(Vpk)
  UWM_controller/2(w) -> microsource/2(w), Gain/1
  Current Measurement/1 -> UWM_controller/2(i_meas), "RMS "/1
  Voltage Measurement/1 -> UWM_controller/1(v_meas), RMS 1/1
  "RMS "/1 -> Product/1
  RMS 1/1 -> Product/2
  Gain/1 -> w/1
  Product/1 -> Pgen/1
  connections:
  Voltage Measurement/LConn2 -- GND/RConn1 -- Parallel RLC Branch2/RConn1 -- microsource/RConn2
  Parallel RLC Branch1/RConn1 -- Voltage Measurement/LConn1 -- Current Measurement/LConn1
  a/RConn1 -- Current Measurement/RConn1
  Parallel RLC Branch/LConn1 -- microsource/RConn1
  Parallel RLC Branch2/LConn1 -- Parallel RLC Branch1/LConn1 -- Parallel RLC Branch/RConn1

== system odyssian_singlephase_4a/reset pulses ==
  Sum : Sum  Inputs=|++  OutDataType=fixdt(1, 16)  OutScaling=2^0
  pulse : Subsystem  mask{tstart=tpulse(1), dt=.1}
  pulse1 : Subsystem  mask{tstart=tpulse(2), dt=.1}
  Out1 : Outport
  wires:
  pulse/1(Out1) -> Sum/1
  pulse1/1(Out1) -> Sum/2
  Sum/1 -> Out1/1

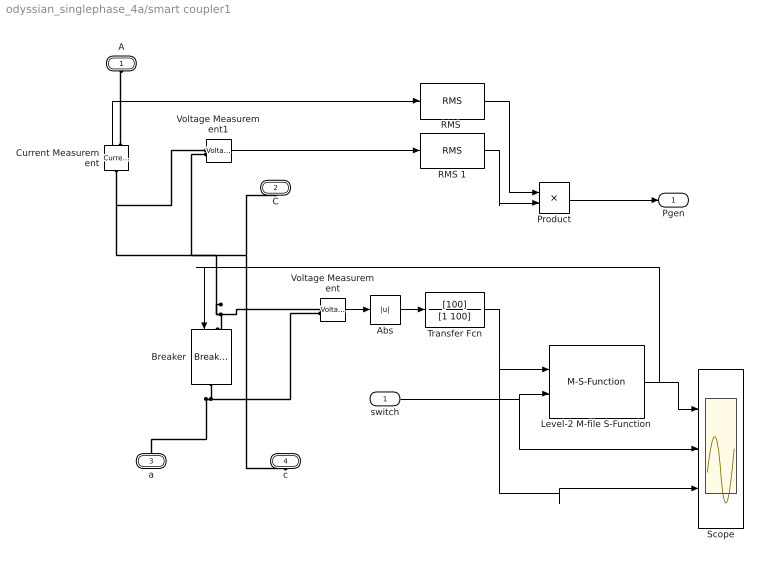
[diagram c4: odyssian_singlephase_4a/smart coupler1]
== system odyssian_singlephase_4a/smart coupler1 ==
  switch : Inport  OutDataType=fixdt(1, 16)  OutScaling=2^0
  Abs : Abs  OutDataType=fixdt(1, 16)  OutScaling=2^0
  Breaker : powerlib/Elements/Breaker  DialogController=POWERSYS.PowerSysDialog  SystemSampleTime=-1  BreakerResistance=0.01  InitialState=0  SnubberResistance=1e6  SnubberCapacitance=inf  SwitchingTimes="[ 1/60  5/60 ]"  External=on  Measurements=None  MoreParameters=off  NoBreakLoop=off
  Current Measurement : powerlib/Measurements/Current Measurement  DialogController=POWERSYS.PowerSysDialog  SystemSampleTime=-1  PhasorSimulation=off  OutputType=Complex  PSBequivalent=0
  Level-2 M-file S-Function : M-S-Function  FunctionName=smart_coupler
  Product : Product  OutDataType=fixdt(1, 16)  OutScaling=2^0
  "RMS " : powerlib_extras/Measurements/RMS  DialogController=POWERSYS.PowerSysDialog  SystemSampleTime=-1  f1=60
  RMS 1 : powerlib_extras/Measurements/RMS  DialogController=POWERSYS.PowerSysDialog  SystemSampleTime=-1  f1=60
  Scope : Scope  NumInputPorts=3
  Transfer Fcn : TransferFcn  Numerator=[100]  Denominator=[1 100]
  Voltage Measurement : powerlib/Measurements/Voltage Measurement  DialogController=POWERSYS.PowerSysDialog  SystemSampleTime=-1  PhasorSimulation=off  OutputType=Complex  PSBequivalent=0
  Voltage Measurement1 : powerlib/Measurements/Voltage Measurement  DialogController=POWERSYS.PowerSysDialog  SystemSampleTime=-1  PhasorSimulation=off  OutputType=Complex  PSBequivalent=0
  A : PMIOPort  Port=1  Side=Left
  C : PMIOPort  Port=2  Side=Left
  a : PMIOPort  Port=3  Side=Right
  c : PMIOPort  Port=4  Side=Right
  Pgen : Outport  OutDataType=fixdt(1, 16)  OutScaling=2^0
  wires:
  switch/1 -> Level-2 M-file S-Function/2, Scope/2
  Level-2 M-file S-Function/1 -> Scope/1, Breaker/1
  Voltage Measurement/1 -> Abs/1
  Abs/1 -> Transfer Fcn/1
  Transfer Fcn/1 -> Level-2 M-file S-Function/1, Scope/3
  "RMS "/1 -> Product/1
  RMS 1/1 -> Product/2
  Product/1 -> Pgen/1
  Current Measurement/1 -> "RMS "/1
  Voltage Measurement1/1 -> RMS 1/1
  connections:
  Breaker/LConn1 -- Current Measurement/LConn1 -- Voltage Measurement1/LConn1 -- Voltage Measurement/LConn1
  Breaker/RConn1 -- Voltage Measurement/LConn2 -- a/RConn1
  c/RConn1 -- C/RConn1 -- Voltage Measurement1/LConn2
  Current Measurement/RConn1 -- A/RConn1

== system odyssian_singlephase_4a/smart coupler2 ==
  switch : Inport  OutDataType=fixdt(1, 16)  OutScaling=2^0
  Abs : Abs  OutDataType=fixdt(1, 16)  OutScaling=2^0
  Breaker : powerlib/Elements/Breaker  DialogController=POWERSYS.PowerSysDialog  SystemSampleTime=-1  BreakerResistance=0.01  InitialState=0  SnubberResistance=1e6  SnubberCapacitance=inf  SwitchingTimes="[ 1/60  5/60 ]"  External=on  Measurements=None  MoreParameters=off  NoBreakLoop=off
  Current Measurement : powerlib/Measurements/Current Measurement  DialogController=POWERSYS.PowerSysDialog  SystemSampleTime=-1  PhasorSimulation=off  OutputType=Complex  PSBequivalent=0
  Level-2 M-file S-Function : M-S-Function  FunctionName=smart_coupler
  Product : Product  OutDataType=fixdt(1, 16)  OutScaling=2^0
  "RMS " : powerlib_extras/Measurements/RMS  DialogController=POWERSYS.PowerSysDialog  SystemSampleTime=-1  f1=60
  RMS 1 : powerlib_extras/Measurements/RMS  DialogController=POWERSYS.PowerSysDialog  SystemSampleTime=-1  f1=60
  Scope : Scope  NumInputPorts=3
  Transfer Fcn : TransferFcn  Numerator=[100]  Denominator=[1 100]
  Voltage Measurement : powerlib/Measurements/Voltage Measurement  DialogController=POWERSYS.PowerSysDialog  SystemSampleTime=-1  PhasorSimulation=off  OutputType=Complex  PSBequivalent=0
  Voltage Measurement1 : powerlib/Measurements/Voltage Measurement  DialogController=POWERSYS.PowerSysDialog  SystemSampleTime=-1  PhasorSimulation=off  OutputType=Complex  PSBequivalent=0
  A : PMIOPort  Port=1  Side=Left
  C : PMIOPort  Port=2  Side=Left
  a : PMIOPort  Port=3  Side=Right
  c : PMIOPort  Port=4  Side=Right
  Pgen : Outport  OutDataType=fixdt(1, 16)  OutScaling=2^0
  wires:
  switch/1 -> Level-2 M-file S-Function/2, Scope/2
  Level-2 M-file S-Function/1 -> Scope/1, Breaker/1
  Voltage Measurement/1 -> Abs/1
  Abs/1 -> Transfer Fcn/1
  Transfer Fcn/1 -> Level-2 M-file S-Function/1, Scope/3
  "RMS "/1 -> Product/1
  RMS 1/1 -> Product/2
  Product/1 -> Pgen/1
  Current Measurement/1 -> "RMS "/1
  Voltage Measurement1/1 -> RMS 1/1
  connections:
  Voltage Measurement/LConn1 -- Breaker/LConn1 -- Current Measurement/LConn1 -- Voltage Measurement1/LConn1
  Breaker/RConn1 -- Voltage Measurement/LConn2 -- a/RConn1
  c/RConn1 -- C/RConn1 -- Voltage Measurement1/LConn2
  Current Measurement/RConn1 -- A/RConn1

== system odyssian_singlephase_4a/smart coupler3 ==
  switch : Inport  OutDataType=fixdt(1, 16)  OutScaling=2^0
  Abs : Abs  OutDataType=fixdt(1, 16)  OutScaling=2^0
  Breaker : powerlib/Elements/Breaker  DialogController=POWERSYS.PowerSysDialog  SystemSampleTime=-1  BreakerResistance=0.01  InitialState=0  SnubberResistance=1e6  SnubberCapacitance=inf  SwitchingTimes="[ 1/60  5/60 ]"  External=on  Measurements=None  MoreParameters=off  NoBreakLoop=off
  Current Measurement : powerlib/Measurements/Current Measurement  DialogController=POWERSYS.PowerSysDialog  SystemSampleTime=-1  PhasorSimulation=off  OutputType=Complex  PSBequivalent=0
  Level-2 M-file S-Function : M-S-Function  FunctionName=smart_coupler
  Product : Product  OutDataType=fixdt(1, 16)  OutScaling=2^0
  "RMS " : powerlib_extras/Measurements/RMS  DialogController=POWERSYS.PowerSysDialog  SystemSampleTime=-1  f1=60
  RMS 1 : powerlib_extras/Measurements/RMS  DialogController=POWERSYS.PowerSysDialog  SystemSampleTime=-1  f1=60
  Scope : Scope  NumInputPorts=3
  Transfer Fcn : TransferFcn  Numerator=[100]  Denominator=[1 100]
  Voltage Measurement : powerlib/Measurements/Voltage Measurement  DialogController=POWERSYS.PowerSysDialog  SystemSampleTime=-1  PhasorSimulation=off  OutputType=Complex  PSBequivalent=0
  Voltage Measurement1 : powerlib/Measurements/Voltage Measurement  DialogController=POWERSYS.PowerSysDialog  SystemSampleTime=-1  PhasorSimulation=off  OutputType=Complex  PSBequivalent=0
  A : PMIOPort  Port=1  Side=Left
  C : PMIOPort  Port=2  Side=Left
  a : PMIOPort  Port=3  Side=Right
  c : PMIOPort  Port=4  Side=Right
  Pgen : Outport  OutDataType=fixdt(1, 16)  OutScaling=2^0
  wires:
  switch/1 -> Level-2 M-file S-Function/2, Scope/2
  Level-2 M-file S-Function/1 -> Scope/1, Breaker/1
  Voltage Measurement/1 -> Abs/1
  Abs/1 -> Transfer Fcn/1
  Transfer Fcn/1 -> Level-2 M-file S-Function/1, Scope/3
  "RMS "/1 -> Product/1
  RMS 1/1 -> Product/2
  Product/1 -> Pgen/1
  Current Measurement/1 -> "RMS "/1
  Voltage Measurement1/1 -> RMS 1/1
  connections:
  Breaker/LConn1 -- Current Measurement/LConn1 -- Voltage Measurement1/LConn1 -- Voltage Measurement/LConn1
  Breaker/RConn1 -- Voltage Measurement/LConn2 -- a/RConn1
  c/RConn1 -- C/RConn1 -- Voltage Measurement1/LConn2
  Current Measurement/RConn1 -- A/RConn1
